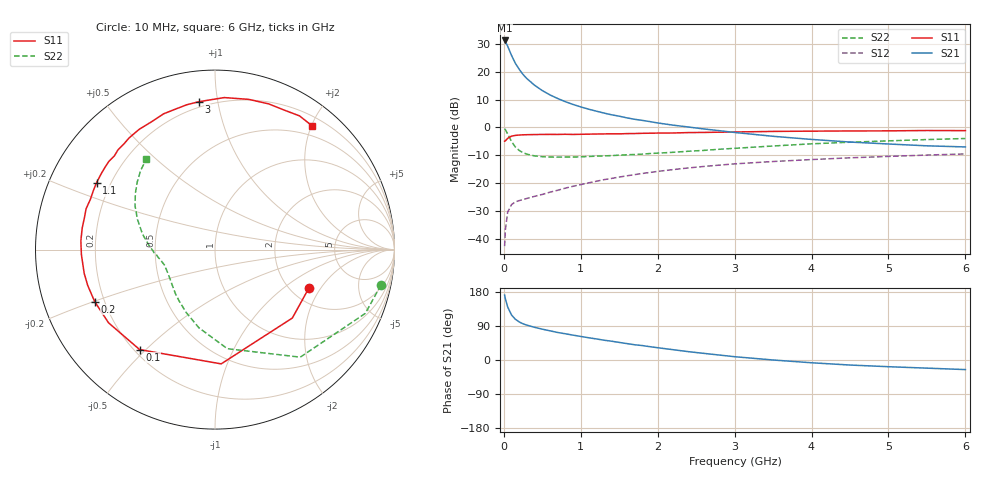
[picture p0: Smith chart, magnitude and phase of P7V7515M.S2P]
! SIEMENS Small Signal Semiconductors
! BFP196
! Si NPN RF Bipolar Junction Transistor in SOT143
! VCE = 0.75 V  IC = 15 mA
! Common Emitter S-Parameters:  May  1996
# GHz  S  MA  R  50
!  f  S11  S21  S12  S22
! GHz  MAG  ANG  MAG  ANG  MAG  ANG  MAG  ANG
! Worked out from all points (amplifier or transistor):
!   36 points, 10 MHz to 6 GHz, reference 50 ohm
!   highest |S21| = 31.3 dB at 10 MHz (marker M1)
!   |S21| within 3 dB of that: start of sweep to 63.99 MHz
!   unconditionally stable (mu >= 1): 695.9 MHz to end of sweep
!   at 250 MHz: K = 0.53, MSG = 22.5 dB, |S12| = -26.0 dB
!   at 1.4 GHz: K = 1.14, MAG = 9.2 dB, |S12| = -18.3 dB
!   at 6 GHz: K = 1.03, MAG = 0.3 dB, |S12| = -9.5 dB
!   S11 on the Smith chart (normalised r, x): 10 MHz: 2.50, -1.56; 100 MHz: 0.22, -0.48; 200 MHz: 0.16, -0.20; 1.1 GHz: 0.15, +0.26; 3 GHz: 0.17, +0.88; 6 GHz: 0.34, +2.00
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0.01  0.5654 -22.1  36.79 171.3  0.0073 81.2  0.9457 -12.0
0.02  0.5754 -41.5  34.92 161.5  0.0144 74.0  0.9097 -23.0
0.05  0.6376 -86.9  28.99 139.9  0.03 55.2  0.7647 -51.6
0.1  0.6976 -127.0  19.78 118.7  0.0409 39.8  0.5564 -82.9
0.15  0.7199 -145.5  14.27 107.5  0.0458 34.5  0.4449 -101.6
0.2  0.7302 -156.6  11.13 100.4  0.0483 32.9  0.3855 -114.6
0.25  0.7368 -164.3  8.979 95.5  0.0503 32.8  0.3499 -124.6
0.3  0.7407 -169.7  7.559 91.9  0.0528 34.4  0.3311 -131.5
0.4  0.7449 -177.9  5.746 86.2  0.0576 36.8  0.3072 -141.6
0.5  0.7489 176.3  4.606 81.4  0.0623 39.2  0.2974 -148.5
0.6  0.7497 170.9  3.85 77.0  0.0684 41.5  0.2937 -153.3
0.7  0.749 166.0  3.317 72.6  0.0741 43.3  0.2927 -156.9
0.9  0.7487 158.0  2.592 65.6  0.0874 45.1  0.2932 -162.1
1.1  0.7577 150.6  2.137 58.8  0.1005 46.2  0.3004 -165.7
1.3  0.7652 143.4  1.819 52.3  0.1148 46.0  0.3073 -169.1
1.6  0.7751 134.2  1.487 43.3  0.1348 44.6  0.3224 -173.1
2.2  0.7949 116.6  1.1 27.2  0.1744 39.1  0.357 178.7
3  0.8288 96.3  0.813 8.7  0.221 29.4  0.421 166.2
3.5  0.8486 86.5  0.693 0.0  0.2439 23.3  0.4637 158.7
4.5  0.8651 69.9  0.546 -13.3  0.2842 12.0  0.5425 144.9
5.5  0.8814 57.7  0.467 -21.5  0.3185 1.4  0.6056 133.1
6  0.8766 52.0  0.446 -25.3  0.3341 -4.5  0.6326 127.2
